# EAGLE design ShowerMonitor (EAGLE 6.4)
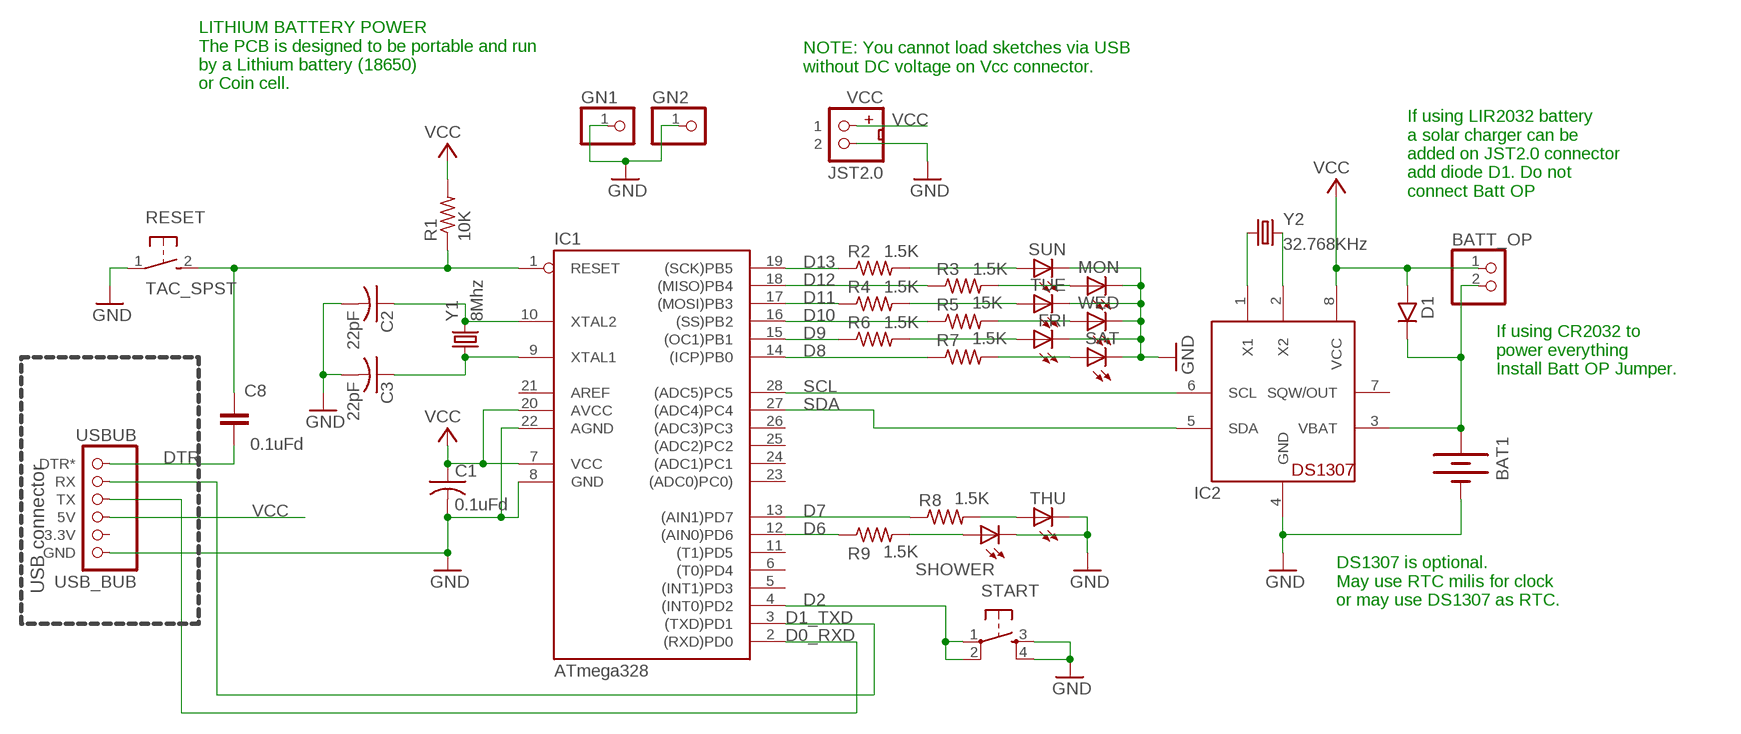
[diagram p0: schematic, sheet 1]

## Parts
BAT1  BATTERY20PTH  [BATTCOM_20MM_PTH]
BATT_OP  PINHD-1X2  [1X02]
C1  0.1uFd  C-US050-024X044  [C050-024X044]
C2  22pF  C-US025-025X050  [C025-025X050]
C3  22pF  C-US025-025X050  [C025-025X050]
C8  0.1uFd  C-EU050-025X075  [C050-025X075]
D1  1N400X.1  [DO41-1]
FRI  LED3MM  [LED3MM]
GN1  PINHD-1X1  [1X01]
GN2  PINHD-1X1  [1X01]
IC1  ATmega328  AT90S4433P  [DIL28-3]
IC2  DS1307  [DIL08]
MON  LED3MM  [LED3MM]
R1  10K  R-US_0207/2V  [0207/2V]
R2  1.5K  R-US_0207/2V  [0207/2V]
R3  1.5K  R-US_0207/2V  [0207/2V]
R4  1.5K  R-US_0207/2V  [0207/2V]
R5  15K  R-US_0207/2V  [0207/2V]
R6  1.5K  R-US_0207/2V  [0207/2V]
R7  1.5K  R-US_0207/2V  [0207/2V]
R8  1.5K  R-US_0207/2V  [0207/2V]
R9  1.5K  R-US_0207/2V  [0207/2V]
RESET  TAC_SPST  [TACTILE-SPST]
SAT  LED3MM  [LED3MM]
SHOWER  LED3MM  [LED3MM]
START  TAC_SWITCHPTH  [TACTILE-PTH]
SUN  LED3MM  [LED3MM]
THU  LED3MM  [LED3MM]
TUE  LED3MM  [LED3MM]
USBUB  USB_BUB  [USB_BUB]
VCC  JST2.0  [JST2.0]
WED  LED3MM  [LED3MM]
Y1  8Mhz  CRYSTALTC38H  [TC38H]
Y2  32.768KHz  CRYSTALTC38H  [TC38H]

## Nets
D0_RXD: IC1.2((RXD)PD0) USBUB.TX
D1_TXD: IC1.3((TXD)PD1) USBUB.RX
D2: IC1.4((INT0)PD2) START.1 START.2
D6: IC1.12((AIN0)PD6) R9.1
D7: IC1.13((AIN1)PD7) R8.1
D8: IC1.14((ICP)PB0) R7.1
D9: IC1.15((OC1)PB1) R6.1
D10: IC1.16((SS)PB2) R5.1
D11: IC1.17((MOSI)PB3) R4.1
D12: IC1.18((MISO)PB4) R3.1
D13: IC1.19((SCK)PB5) R2.1
DTR: C8.1 USBUB.DTR*
GND [power]: BAT1.2(-) C1.2 C2.2 C3.2 FRI.K(C) GN1.1 GN2.1 IC1.8(GND) IC1.22(AGND) IC2.4(GND) MON.K(C) RESET.1 SAT.K(C) SHOWER.K(C) START.3 START.4 SUN.K(C) THU.K(C) TUE.K(C) USBUB.GND VCC.2 WED.K(C)
N$1: R2.2 SUN.A
N$2: R8.2 THU.A
N$3: MON.A R3.2
N$4: R4.2 TUE.A
N$5: R5.2 WED.A
N$6: C3.1 IC1.9(XTAL1) Y1.1
N$7: C2.1 IC1.10(XTAL2) Y1.2
N$8: FRI.A R6.2
N$9: R7.2 SAT.A
N$10: IC2.1(X1) Y2.1
N$11: IC2.2(X2) Y2.2
N$12: R9.2 SHOWER.A
RESET: C8.2 IC1.1(RESET) R1.1 RESET.2
SCL: IC1.28((ADC5)PC5) IC2.6(SCL)
SDA: IC1.27((ADC4)PC4) IC2.5(SDA)
VBAT: BAT1.1(+) BATT_OP.2 D1.C IC2.3(VBAT)
VCC: BATT_OP.1 C1.1 D1.A IC1.7(VCC) IC1.20(AVCC) IC2.8(VCC) R1.2 USBUB.5V VCC.1
Unconnected: IC1.5((INT1)PD3) IC1.6((T0)PD4) IC1.11((T1)PD5) IC1.21(AREF) IC1.23((ADC0)PC0)) IC1.24((ADC1)PC1) IC1.25((ADC2)PC2) IC1.26((ADC3)PC3) IC2.7(SQW/OUT) USBUB.3.3V

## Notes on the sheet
- NOTE: You cannot load sketches via USB 
  without DC voltage on Vcc connector.
- LITHIUM BATTERY POWER
  The PCB is designed to be portable and run
  by a Lithium battery (18650)
  or Coin cell.
- If using LIR2032 battery
  a solar charger can be
  added on JST2.0 connector
  add diode D1. Do not
  connect Batt OP
- If using CR2032 to
  power everything
  Install Batt OP Jumper.
- USB connector
- DS1307 is optional. 
  May use RTC milis for clock 
  or may use DS1307 as RTC.

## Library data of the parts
BAT1 = SparkFun:BATTERY: Battery Holders
BATT_OP = MTS_Custom:PINHD-1X2: PIN HEADER
C1-C3 = MTS:C-US: CAPACITOR, American symbol
C8 = my-rcl:C-EU: CAPACITOR, European symbol
D1 = gm-diodes:1N400X: Rectifier Diodes
FRI MON SAT SHOWER SUN THU TUE WED = adafruit:LED: LED
GN1 GN2 = pinhead:PINHD-1X1: PIN HEADER
IC1 = atmel:AT90S4433: MICROCONTROLLER 4 Kbytes FLASH 128 bytes SRAM 256 bytes EEPROM UART 6-channel 10 bit ADC
IC2 = adafruit:DS1307: DS1307 Real time clock (RTC) with battery backup ability. Talk to it via i2c
R1-R9 = MTS:R-US_: RESISTOR, American symbol
RESET = MTS_Custom:TAC_SPST: Tactile switch SPST 7mm lead spacing
START = SparkFun:TAC_SWITCH: Momentary Switch Button commonly used for reset or general input. Spark Fun Electronics SKU : COM-00097
USBUB = MTS:USB_BUB
VCC = MTS_Custom:JST2.0
Y1 = MTS:CRYSTAL: Crystals
Y2 = SparkFun:CRYSTAL: Crystals

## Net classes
0 default: width 0.4 mm, clearance 0.3 mm
1 power: width 0.6 mm, clearance 0.3 mm

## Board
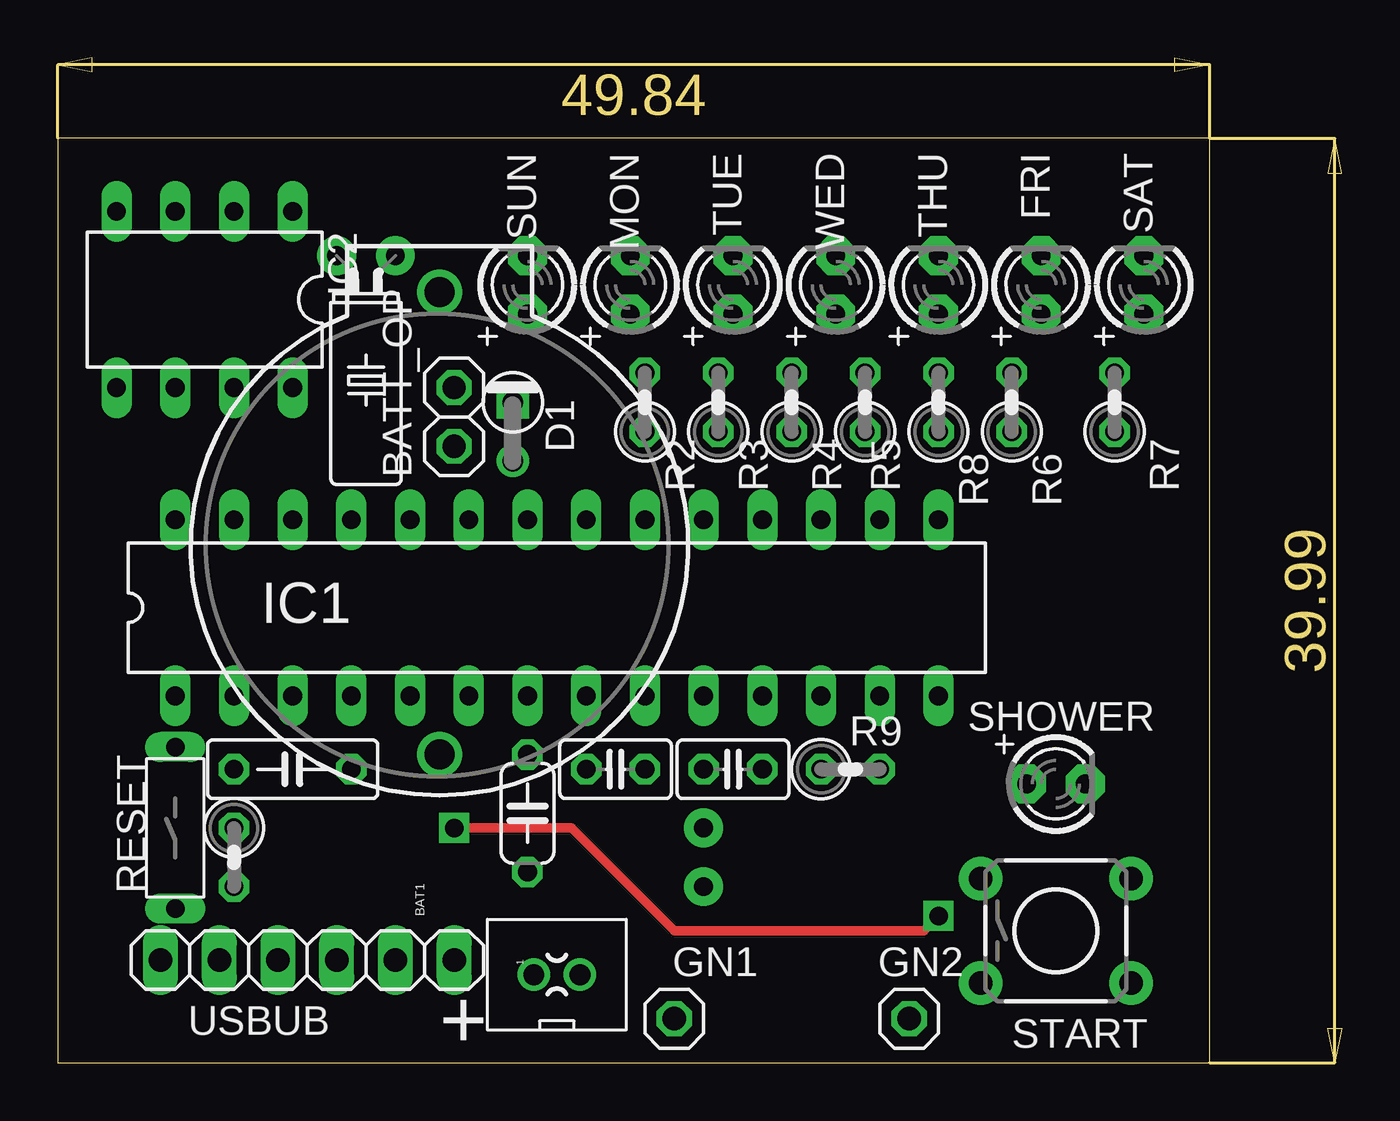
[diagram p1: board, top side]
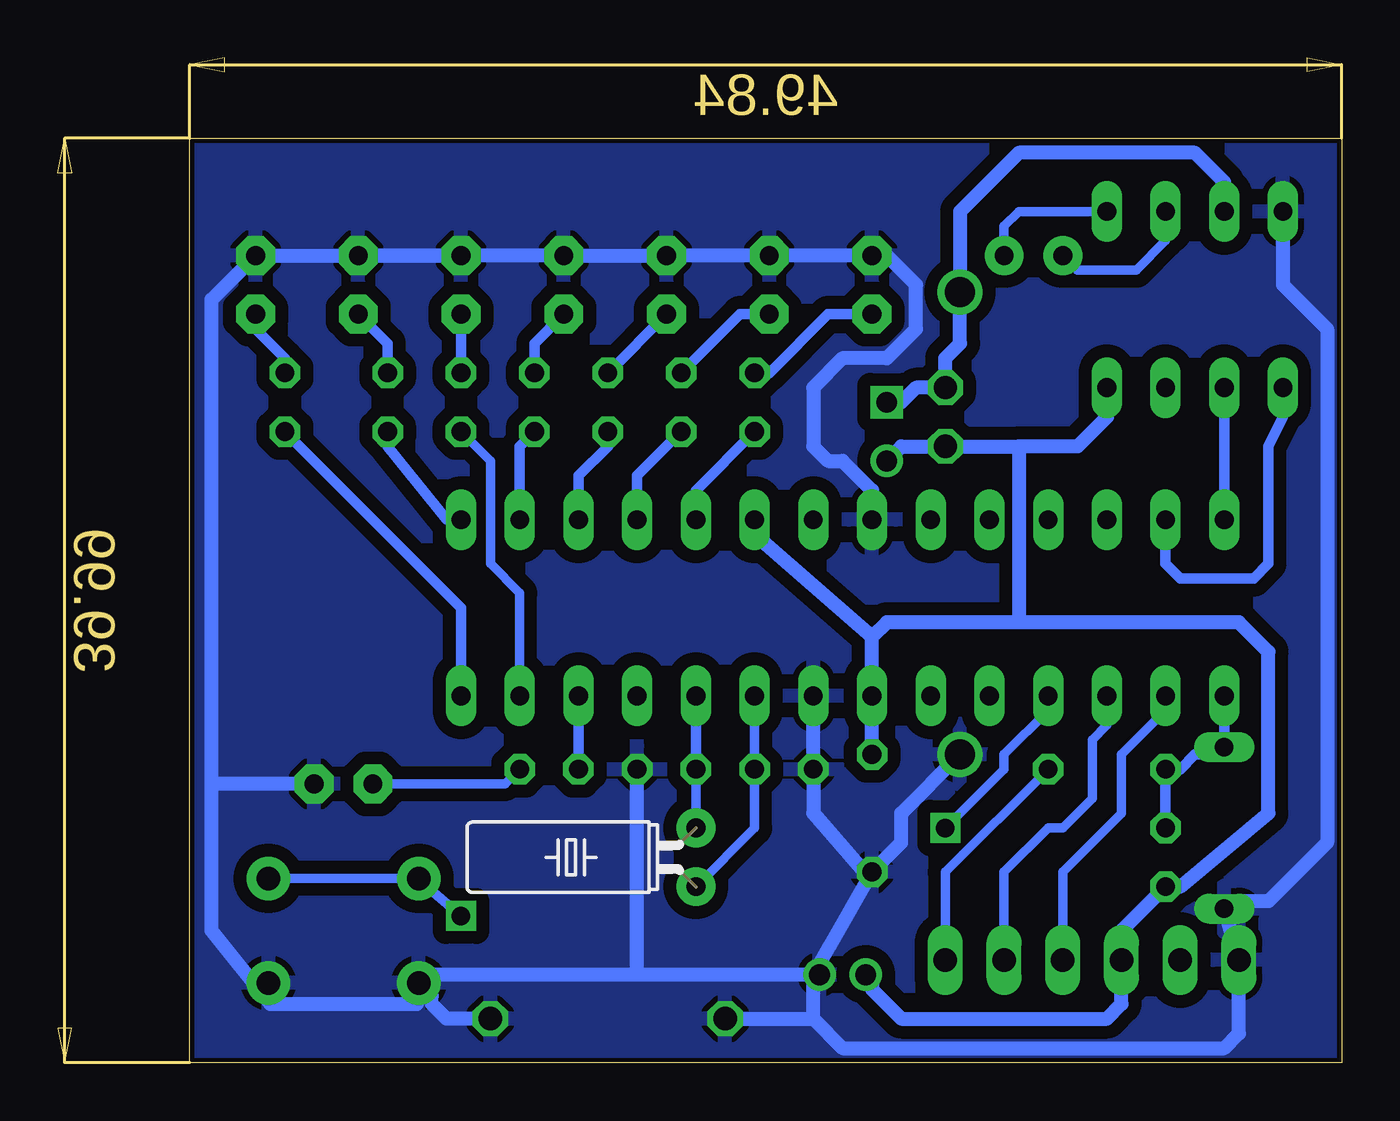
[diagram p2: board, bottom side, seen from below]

Size 55.54 x 43.48 mm. Coordinates in mm from the lower left corner, seen from the top.
Outline: 0,0 49.84,0 49.84,39.99 0,39.99 0,0
Copper layers (1*16): Top 0.035mm / dielectric 1.5mm / Bottom 0.035mm
Design rules "MTS1 *": minimum track width 18mil, minimum drill 12mil, track to track 22mil, track to pad 22mil, pad to pad 6mil, via to via 6mil, smd to smd 0mil, copper to edge 8mil, drill to drill 10mil, minimum pad ring 10mil, minimum via ring 10mil, stop-mask expansion 2mil, vias tented up to drill 25mil, thermal gap 10mil

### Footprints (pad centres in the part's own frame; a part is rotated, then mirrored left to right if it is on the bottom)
BATTCOM_20MM_PTH = drill 1.3: 1 20,0; 2 0,0
1X02 = drill 1 octagon: 1 -1.27,0; 2 1.27,0
C050-024X044 = drill 0.813 octagon: 1 -2.54,0; 2 2.54,0
C025-025X050 = drill 0.813 octagon: 1 -1.27,0; 2 1.27,0
C050-025X075 = drill 0.813 octagon: 1 -2.54,0; 2 2.54,0
DO41-1 = drill 0.9: A 1.27,0 | drill 0.9 square: C -1.27,0
LED3MM = drill 0.813 pad 1.676 octagon: A -1.27,0; K 1.27,0
1X01 = drill 1.016 octagon: 1 0,0
DIL28-3 = drill 0.813 long: 1 -16.51,-3.81; 2 -13.97,-3.81; 3 -11.43,-3.81; 4 -8.89,-3.81; 5 -6.35,-3.81; 6 -3.81,-3.81; 7 -1.27,-3.81; 8 1.27,-3.81; 9 3.81,-3.81; 10 6.35,-3.81; 11 8.89,-3.81; 12 11.43,-3.81; 13 13.97,-3.81; 14 16.51,-3.81; 15 16.51,3.81; 16 13.97,3.81; 17 11.43,3.81; 18 8.89,3.81; 19 6.35,3.81; 20 3.81,3.81; 21 1.27,3.81; 22 -1.27,3.81; 23 -3.81,3.81; 24 -6.35,3.81; 25 -8.89,3.81; 26 -11.43,3.81; 27 -13.97,3.81; 28 -16.51,3.81
DIL08 = drill 0.813 long: 1 -3.81,-3.81; 2 -1.27,-3.81; 3 1.27,-3.81; 4 3.81,-3.81; 5 3.81,3.81; 6 1.27,3.81; 7 -1.27,3.81; 8 -3.81,3.81
0207/2V = drill 0.813 octagon: 1 -1.27,0; 2 1.27,0
TACTILE-SPST = drill 0.8 long: 1 0,3.5; 2 0,-3.5
TACTILE-PTH = drill 1.016 pad 1.88: 1 -3.251,2.261; 2 3.251,2.261; 3 -3.251,-2.261; 4 3.251,-2.261
USB_BUB = drill 1.016 long: 3.3V -3.81,0; 5V -1.27,0; DTR* 6.35,0; GND -6.35,0; RX 3.81,0; TX 1.27,0
JST2.0 = drill 0.9 pad 1.016: 1 0,-1; 2 0,1
TC38H = drill 0.813 pad 1.676: 1 -1.27,0; 2 1.27,0

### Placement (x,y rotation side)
BAT1  16.51,13.34 90 top
BATT_OP  17.14,27.94 90 top
C1  20.32,10.79 270 top
C2  29.21,12.7 0 top
C3  24.13,12.7 180 top
C8  10.16,12.7 180 top
D1  19.68,27.3 270 top
FRI  42.55,33.66 90 top
GN1  26.67,1.91 0 top
GN2  36.83,1.91 0 top
IC1  21.59,19.68 0 top
IC2  6.35,33.02 180 top
MON  24.77,33.66 90 top
R1  7.62,8.89 270 top
R2  25.4,28.57 90 top
R3  28.57,28.57 90 top
R4  31.75,28.57 90 top
R5  34.92,28.57 90 top
R6  41.27,28.57 90 top
R7  45.72,28.57 90 top
R8  38.1,28.57 90 top
R9  34.29,12.7 0 top
RESET  5.08,10.16 180 top
SAT  46.99,33.66 90 top
SHOWER  43.18,12.06 0 top
START  43.18,5.71 0 top
SUN  20.32,33.66 90 top
THU  38.1,33.66 90 top
TUE  29.21,33.66 90 top
USBUB  10.79,4.45 0 top
VCC  21.59,3.81 270 top
WED  33.66,33.66 90 top
Y1  27.94,8.89 90 bottom
Y2  13.34,34.92 180 top

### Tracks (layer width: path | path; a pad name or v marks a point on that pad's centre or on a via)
D0_RXD
  Bottom 0.406: IC1.2 7.62,15.24 9.53,13.34 9.53,10.79 12.06,8.26 USBUB.TX
D1_TXD
  Bottom 0.406: IC1.3 10.16,14.61 10.79,13.97 10.79,11.43 12.06,10.16 12.7,10.16 14.61,8.26 USBUB.RX
D2  (via drill 0.8)
  Top 0.406: v17.14,10.16 22.23,10.16 26.67,5.71 37.47,5.71 v38.1,6.35
  Bottom 0.406: IC1.4 12.7,15.24 14.61,13.34 14.61,12.7 v17.14,10.16 | v38.1,6.35 39.57,7.62 START.1 START.2
D6
  Bottom 0.457: R9.1 IC1.12
D7
  Bottom 0.406: IC1.13 35.56,20.32 36.83,21.59 36.83,26.04 R8.1
D8
  Bottom 0.457: R7.1 38.1,19.68 IC1.14
D9
  Bottom 0.457: R6.1 41.27,26.67 38.73,23.5 IC1.15
D10
  Bottom 0.457: R5.1 35.56,26.67 IC1.16
D11
  Bottom 0.457: IC1.17 33.02,25.4 31.75,26.67 R4.1
D12
  Bottom 0.457: R3.1 30.48,25.4 IC1.18
D13
  Bottom 0.457: IC1.19 27.94,24.77 R2.1
DTR
  Bottom 0.406: C8.1 17.14,8.26 USBUB.DTR*
GND
  Bottom 0.6: IC1.8 C3.2 22.86,10.79 20.75,8.37 C1.2 | FRI.K THU.K | 19.68,34.92 SUN.K MON.K TUE.K WED.K FRI.K | IC1.22 20.32,24.77 21.59,26.04 22.23,26.04 22.86,26.67 22.86,29.21 21.59,30.48 19.68,30.48 18.41,31.75 | C1.2 22.16,5.04 22.86,3.81 | RESET.1 USBUB.GND 4.45,1.27 5.08,0.64 21.59,0.64 22.86,1.91 22.86,3.81 | 22.86,3.81 VCC.2 | FRI.K SAT.K 48.9,33.02 48.9,12.06 48.9,5.71 46.35,2.54 | C1.2 19.05,9.53 19.05,10.79 BAT1.2 | 46.35,2.54 40.01,2.54 START.3 39.37,3.81 30.48,3.81 | 46.35,2.54 START.4 | 30.48,3.81 C2.2 | 22.86,3.81 30.48,3.81
  Bottom 0.61: IC2.4 2.54,33.66 0.64,31.75 0.64,9.53 3.17,6.99 4.75,6.99 RESET.1 | SHOWER.K 48.9,12.06 | GN2.1 38.73,1.91 39.37,2.54 39.37,2.9 START.3 | GN1.1 22.86,1.91 | 18.41,31.75 18.41,33.66 19.68,34.92
  pour Bottom: 0,0 50.8,0 50.8,40.64 0,40.64
N$1
  Bottom 0.457: SUN.A 22.23,32.38 24.77,29.84 R2.2
N$2
  Bottom 0.457: THU.A R8.2
N$3
  Bottom 0.457: R3.2 26.04,32.38 MON.A
N$4
  Bottom 0.457: TUE.A R4.2
N$5
  Bottom 0.457: R5.2 34.92,31.11 WED.A
N$6
  Bottom 0.406: IC1.9 C3.1 25.4,10.16 Y1.1
N$7
  Bottom 0.406: C2.1 Y1.2
  Bottom 0.457: C2.1 IC1.10
N$8
  Bottom 0.457: R6.2 41.27,31.11 FRI.A
N$9
  Bottom 0.457: R7.2 45.72,30.48 46.99,31.75 SAT.A
N$10
  Bottom 0.406: Y2.1 14.61,36.2 13.97,36.83 IC2.1
N$11
  Bottom 0.406: Y2.2 11.43,34.29 8.89,34.29 7.62,35.56 IC2.2
N$12
  Bottom 0.406: R9.2 36.2,12.06 SHOWER.A
RESET
  Bottom 0.457: R1.1 C8.2 6.99,12.7 6.35,13.34 5.08,13.34 RESET.2 IC1.1
SCL
  Bottom 0.457: IC2.6 IC1.28
SDA
  Bottom 0.457: IC2.5 2.54,27.94 3.17,26.67 3.17,21.59 3.81,20.95 6.99,20.95 7.62,21.59 IC1.27
VBAT
  Bottom 0.61: IC2.3 5.08,38.1 6.35,39.37 13.97,39.37 16.51,36.83 BAT1.1 16.51,31.11 17.14,30.48 BATT_OP.2 18.41,29.21 19.05,28.57 D1.C
VCC
  Bottom 0.61: 20.32,18.41 IC1.7 C1.1 | 20.32,18.41 25.4,22.86 IC1.20 | 13.97,19.05 4.45,19.05 3.17,17.78 3.17,10.79 6.99,7.62 R1.2 9.53,5.71 USBUB.5V 9.53,2.54 10.16,1.91 19.05,1.91 20.32,3.17 20.32,3.81 VCC.1 | 13.97,19.05 19.68,19.05 20.32,18.41 | IC2.8 10.16,27.94 11.43,26.67 13.97,26.67 | 13.97,26.67 BATT_OP.1 19.05,26.67 D1.A | 13.97,26.67 13.97,19.05

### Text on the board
tNames: +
